|   IBIS file stm32l471_476_ufbga144.ibs
[IBIS ver]   4.2
[File name]   stm32l471_476_ufbga144.ibs
[File Rev]   1.0
[Date]   08-10-2018
[Source]   Data Created at STMicroelectronics
[Notes]   File originated from ELDO simulations.
[Disclaimer]  This information is for modeling purpose only and is
   not guaranteed.
   The information is subject to change without notice.
[Copyright]   Copyright 2018 STMicroelectronics Inc.
|   Component stm32l471_476_ufbga144
[Component] stm32l471_476_ufbga144
[Manufacturer] STMicroelectronics
[Package]
| variable   typ   min   max
R_pkg   0.0   0.0   0.0
L_pkg   0.0H   0.0H   0.0H
C_pkg   0.0F   0.0F   0.0F
[Pin]  signal_name   model_name   R_pin   L_pin   C_pin
A1 VSS GND
A10 PD1 io8prog2m25m50m120m_sudq_ft
A11 PD0 io8prog2m25m50m120m_sudq_ft
A12 VSS GND
A2 PE0 io8prog2m25m50m120m_sudq_ft
A3 PB8 io8prog2m25m50m120m_sudq_i2c_ft
A4 BOOT0 vpp_test_hv
A5 PB7 io8prog2m25m50m120m_sudq_i2c_ft
A6 PG14 io8prog2m25m50m120m_sudq_i2c_ft
A7 PG12 io8prog2m25m50m120m_sudq_ft
A8 PD7 io8prog2m25m50m120m_sudq_ft
A9 PD6 io8prog2m25m50m120m_sudq_ft
B1 VBAT POWER
B10 PC10 io8prog2m25m50m120m_sudq_ft
B11 PA12 io8usblsfs_otg2
B12 PA11 io8usblsfs_otg2
B2 PE4 io8prog2m25m50m120m_sudq_ft
B3 PE3 io8prog2m25m50m120m_sudq_ft
B4 PE1 io8prog2m25m50m120m_sudq_ft
B5 PB6 io8prog2m25m50m120m_sudq_i2c_ft
B6 PG15 io8prog2m25m50m120m_sudq_ft
B7 PG11 io8prog2m25m50m120m_sudq_ft
B8 PD5 io8prog2m25m50m120m_sudq_ft
B9 PC12 io8prog2m25m50m120m_sudq_ft
C1 PC15-OSC32_OUT io8prog2m25m50m120m_sudq_ft
C10 PA14 io8prog2m25m50m120m_sudq_ft
C11 PA13 io8prog2m25m50m120m_sudq_ft
C12 PA10 io8usb_id_otg20_lcd4_ft_ms
C2 PE5 io8prog2m25m50m120m_sudq_ft
C3 PE2 io8prog2m25m50m120m_sudq_ft
C4 PB9 io8prog2m25m50m120m_sudq_i2c_ft
C5 PB5 io8prog2m25m50m120m_sudq_ft
C6 PB3 io8prog2m25m50m120m_sudq_ft
C7 PG9 io8prog2m25m50m120m_sudq_ft
C8 PD4 io8prog2m25m50m120m_sudq_ft
C9 PC11 io8prog2m25m50m120m_sudq_ft
D1 PF4 io8prog2m25m50m120m_sudq_ft
D10 PA15 io8prog2m25m50m120m_sudq_ft
D11 PA9 POWER
D12 PA8 io8prog2m25m50m120m_sudq_ft
D2 PC14-OSC32_IN io8prog2m25m50m120m_sudq_ft
D3 PE6 io8prog2m25m50m120m_sudq_ft
D4 PC13 io8prog2m25m50m120m_sudq_ft
D5 PB4 io8prog2m25m50m120m_sudq_ft
D6 PG13 io8prog2m25m50m120m_sudq_i2c_ft
D7 PG10 io8prog2m25m50m120m_sudq_ft
D8 PD3 io8prog2m25m50m120m_sudq_ft
D9 PD2 io8prog2m25m50m120m_sudq_ft
E1 PF6 io8prog2m25m50m120m_sudq_ft
E10 PC6 io8prog2m25m50m120m_sudq_ft
E11 PC9 io8prog2m25m50m120m_sudq_ft
E12 PC8 io8prog2m25m50m120m_sudq_ft
E2 PF1 io8prog2m25m50m120m_sudq_i2c_ft
E3 PF0 io8prog2m25m50m120m_sudq_i2c_ft
E4 PF2 io8prog2m25m50m120m_sudq_ft
E5 VSS GND
E6 VDDIO2 POWER
E7 VDD POWER
E8 VSS GND
E9 VDD/VDDUSB POWER
F1 PF8 io8prog2m25m50m120m_sudq_ft
F10 PG6 io8prog2m25m50m120m_sudq_ft
F11 PG8 io8prog2m25m50m120m_sudq_i2c_ft
F12 PC7 io8prog2m25m50m120m_sudq_ft
F2 PF7 io8prog2m25m50m120m_sudq_ft
F3 PF5 io8prog2m25m50m120m_sudq_ft
F4 PF3 io8prog2m25m50m120m_sudq_ft
F5 VDD POWER
F6 VSS GND
F7 VSS GND
F8 VDDIO2 POWER
F9 PG7 io8prog2m25m50m120m_sudq_i2c_ft
G1 PH1-OSC_OUT io8prog2m25m50m120m_sudq_ft
G10 PD13 io8prog2m25m50m120m_sudq_ft
G11 PG3 io8prog2m25m50m120m_sudq_ft
G12 PG5 io8prog2m25m50m120m_sudq_ft
G2 PH0-OSC_IN io8prog2m25m50m120m_sudq_ft
G3 PF10 io8prog2m25m50m120m_sudq_ft
G4 PF9 io8prog2m25m50m120m_sudq_ft
G5 VDD POWER
G6 VSS GND
G7 VSS GND
G8 VDD POWER
G9 PG4 io8prog2m25m50m120m_sudq_ft
H1 PC2 io8prog2m25m50m120m_sudq_ft
H10 PD11 io8prog2m25m50m120m_sudq_ft
H11 PD14 io8prog2m25m50m120m_sudq_ft
H12 PG2 io8prog2m25m50m120m_sudq_ft
H2 PC0 io8prog2m25m50m120m_sudq_i2c_ft
H3 PC1 io8prog2m25m50m120m_sudq_i2c_ft
H4 NRST ioreset_ft_v33
H5 VSS GND
H6 VDD POWER
H7 VDD POWER
H8 VSS GND
H9 PD12 io8prog2m25m50m120m_sudq_ft
J1 VSSA GND
J10 PB14 io8prog2m25m50m120m_sudq_i2c_ft
J11 PD10 io8prog2m25m50m120m_sudq_ft
J12 PD15 io8prog2m25m50m120m_sudq_ft
J2 VREF- POWER
J3 PA0 io8prog2m25m50m120m_sudq_ft
J4 PC3 io8prog2m25m50m120m_sudq_ft
J5 PC4 io8prog2m25m50m120m_sudq_ft
J6 PF11 io8prog2m25m50m120m_sudq_ft
J7 PG1 io8prog2m25m50m120m_sudq_ft
J8 PE9 io8prog2m25m50m120m_sudq_ft
J9 PB13 io8prog2m25m50m120m_sudq_i2c_ft
K1 VREF+ POWER
K10 PB12 io8w_swp_lcd4_ft
K11 PD8 io8prog2m25m50m120m_sudq_ft
K12 PD9 io8prog2m25m50m120m_sudq_ft
K2 VDDA POWER
K3 PA1 io8prog2m25m50m120m_sudq_ft
K4 PA6 io8prog2m25m50m120m_sudq_ft
K5 PB2 io8prog2m25m50m120m_sudq_ft
K6 PF12 io8prog2m25m50m120m_sudq_ft
K7 PG0 io8prog2m25m50m120m_sudq_ft
K8 PE11 io8prog2m25m50m120m_sudq_ft
K9 PB11 io8prog2m25m50m120m_sudq_i2c_ft
L1 OPAMP1_VINM NC
L10 PE14 io8prog2m25m50m120m_sudq_ft
L11 PB10 io8prog2m25m50m120m_sudq_i2c_ft
L12 PB15 io8prog2m25m50m120m_sudq_ft
L2 PA2 io8prog2m25m50m120m_sudq_ft
L3 PA4 io8prog2m25m50m120m_sudq_ft
L4 OPAMP2_VINM NC
L5 PB0 io8prog2m25m50m120m_sudq_ft
L6 PF13 io8prog2m25m50m120m_sudq_ft
L7 PE8 io8prog2m25m50m120m_sudq_ft
L8 PE12 io8prog2m25m50m120m_sudq_ft
L9 PE13 io8prog2m25m50m120m_sudq_ft
M1 VSS GND
M10 PE10 io8prog2m25m50m120m_sudq_ft
M11 PE15 io8prog2m25m50m120m_sudq_ft
M12 VSS GND
M2 PA3 io8prog2m25m50m120m_sudq_ft
M3 PA5 io8prog2m25m50m120m_sudq_ft
M4 PA7 io8prog2m25m50m120m_sudq_ft
M5 PC5 io8prog2m25m50m120m_sudq_ft
M6 PB1 io8prog2m25m50m120m_sudq_ft
M7 PF14 io8prog2m25m50m120m_sudq_ft
M8 PE7 io8prog2m25m50m120m_sudq_ft
M9 PF15 io8prog2m25m50m120m_sudq_ft
[Model Selector] io8prog2m25m50m120m_sudq_ft
iols8p_sudq_ft_pd_lv  "IO low speed, PD=40kOhm - 1P8V"
iols8p_sudq_ft_pu_lv  "IO low speed, PU=40kOhm - 1P8V"
iols8p_sudq_ft_lv  "IO low speed - 1P8V"
iols8p_sudq_ft_pd  "IO low speed, PD=40kOhm - 3P3V"
iols8p_sudq_ft_pu  "IO low speed, PU=40kOhm - 3P3V"
iols8p_sudq_ft  "IO low speed - 3P3V"
iofs8p_sudq_ft_pd_lv  "IO full speed, PD=40kOhm - 1P8V"
iofs8p_sudq_ft_pu_lv  "IO full speed, PU=40kOhm - 1P8V"
iofs8p_sudq_ft_lv  "IO full speed - 1P8V"
iofs8p_sudq_ft_pd  "IO full speed, PD=40kOhm - 3P3V"
iofs8p_sudq_ft_pu  "IO full speed, PU=40kOhm - 3P3V"
iofs8p_sudq_ft  "IO full speed - 3P3V"
ioms8p_sudq_ft_pd_lv  "IO medium speed, PD=40kOhm - 1P8V"
ioms8p_sudq_ft_pu_lv  "IO medium speed, PU=40kOhm - 1P8V"
ioms8p_sudq_ft_lv  "IO medium speed - 1P8V"
ioms8p_sudq_ft_pd  "IO medium speed, PD=40kOhm - 3P3V"
ioms8p_sudq_ft_pu  "IO medium speed, PU=40kOhm - 3P3V"
ioms8p_sudq_ft  "IO medium speed - 3P3V"
iohs8p_sudq_ft_pd_lv  "IO high speed, PD=40kOhm - 1P8V"
iohs8p_sudq_ft_pu_lv  "IO high speed, PU=40kOhm - 1P8V"
iohs8p_sudq_ft_lv  "IO high speed - 1P8V"
iohs8p_sudq_ft_pd  "IO high speed, PD=40kOhm - 3P3V"
iohs8p_sudq_ft_pu  "IO high speed, PU=40kOhm - 3P3V"
iohs8p_sudq_ft  "IO high speed - 3P3V"
[Model Selector] io8prog2m25m50m120m_sudq_i2c_ft
io8prog_1v8_i2c_pd  "5V Tol GPIO 1.8V range i2c functionality with pull down"
io8prog_1v8_i2c_pu  "5V Tol GPIO 1.8V range i2c functionality with pull up"
io8prog_1v8_i2c  "5V Tol GPIO 1.8V range i2c functionality"
io8prog_3v3_i2c_pd  "5V Tol GPIO 3.3V range i2c functionality with pull down"
io8prog_3v3_i2c_pu  "5V Tol GPIO 3.3V range i2c functionality with pull up"
io8prog_3v3_i2c  "5V Tol GPIO 3.3V range i2c functionality"
io8ls_1v8_pd  "5V Tol GPIO 1.8V range with pd io low speed"
io8ls_1v8_pu  "5V Tol GPIO 1.8V range with pu io low speed"
io8ls_1v8  "5V Tol GPIO 1.8V range io low speed"
io8ls_3v3_pd  "5V Tol GPIO 3.3V range with pd io low speed"
io8ls_3v3_pu  "5V Tol GPIO 3.3V range with pu io low speed"
io8ls_3v3  "5V Tol GPIO 3.3V range io low speed"
io8fs_1v8_pd  "5V Tol GPIO 1.8V range with pd io full speed"
io8fs_1v8_pu  "5V Tol GPIO 1.8V range with pu io full speed"
io8fs_1v8  "5V Tol GPIO 1.8V range io full speed"
io8fs_3v3_pd  "5V Tol GPIO 3.3V range with pd io full speed"
io8fs_3v3_pu  "5V Tol GPIO 3.3V range with pu io full speed"
io8fs_3v3  "5V Tol GPIO 3.3V range io full speed"
io8ms_1v8_pd  "5V Tol GPIO 1.8V range with pd io medium speed"
io8ms_1v8_pu  "5V Tol GPIO 1.8V range with pu io medium speed"
io8ms_1v8  "5V Tol GPIO 1.8V range io medium speed"
io8ms_3v3_pd  "5V Tol GPIO 3.3V range with pd io medium speed"
io8ms_3v3_pu  "5V Tol GPIO 3.3V range with pu io medium speed"
io8ms_3v3  "5V Tol GPIO 3.3V range io medium speed"
io8hs_1v8_pd  "5V Tol GPIO 1.8V range with pd io high speed"
io8hs_1v8_pu  "5V Tol GPIO 1.8V range with pu io high speed"
io8hs_1v8  "5V Tol GPIO 1.8V range io high speed"
io8hs_3v3_pd  "5V Tol GPIO 3.3V range with pd io high speed"
io8hs_3v3_pu  "5V Tol GPIO 3.3V range with pu io high speed"
io8hs_3v3  "5V Tol GPIO 3.3V range io high speed"
[Model Selector] io8usb_id_otg20_lcd4_ft_ms
io8usbid_1v8_id_pu  "ID 1V8 range with pull up"
io8usbid_3v3_id_pu  "ID 3V3 range with pull up"
io8usbid_1v8_id  "ID 1V8 range"
io8usbid_3v3_id  "ID 3V3 range"
io8lsusbid_1v8_pd  "GPIO 1.8V range with pd io low speed"
io8lsusbid_1v8_pu  "GPIO 1.8V range with pu io low speed"
io8lsusbid_1v8  "GPIO 1.8V range io low speed"
io8lsusbid_3v3_pd  "GPIO 3.3V range with pd io low speed"
io8lsusbid_3v3_pu  "GPIO 3.3V range with pu io low speed"
io8lsusbid_3v3  "GPIO 3.3V range io low speed"
io8fsusbid_1v8_pd  "GPIO 1.8V range with pd io full speed"
io8fsusbid_1v8_pu  "GPIO 1.8V range with pu io full speed"
io8fsusbid_1v8  "GPIO 1.8V range io full speed"
io8fsusbid_3v3_pd  "GPIO 3.3V range with pd io full speed"
io8fsusbid_3v3_pu  "GPIO 3.3V range with pu io full speed"
io8fsusbid_3v3  "GPIO 3.3V range io full speed"
io8msusbid_1v8_pd  "GPIO 1.8V range with pd io medium speed"
io8msusbid_1v8_pu  "GPIO 1.8V range with pu io medium speed"
io8msusbid_1v8  "GPIO 1.8V range io medium speed"
io8msusbid_3v3_pd  "GPIO 3.3V range with pd io medium speed"
io8msusbid_3v3_pu  "GPIO 3.3V range with pu io medium speed"
io8msusbid_3v3  "GPIO 3.3V range io medium speed"
io8hsusbid_1v8_pd  "GPIO 1.8V range with pd io high speed"
io8hsusbid_1v8_pu  "GPIO 1.8V range with pu io high speed"
io8hsusbid_1v8  "GPIO 1.8V range io high speed"
io8hsusbid_3v3_pd  "GPIO 3.3V range with pd io high speed"
io8hsusbid_3v3_pu  "GPIO 3.3V range with pu io high speed"
io8hsusbid_3v3  "GPIO 3.3V range io high speed"
[Model Selector] io8usblsfs_otg2
usb_ls_pd  "USB Low Speed mode - Pull Down"
usb_ls_pu2  "USB Low Speed mode - Pull up 2"
usb_ls_pu  "USB Low Speed mode - Pull up"
usb_fs  "USB Low Speed mode"
usb_fs_pd  "USB Full Speed mode - Pull Down"
usb_fs_pu2  "USB Full Speed mode - Pull up 2"
usb_fs_pu  "USB Full Speed mode - Pull up"
[Model Selector] ioreset_ft_v33
ioreset_1v2_pu  "RESET 1.2V range with PU"
ioreset_1v2  "RESET 1.2V range"
ioreset_1v8_pu  "RESET 1.8V range with PU"
ioreset_1v8  "RESET 1.8V range"
ioreset_3v3_pu  "RESET 3.3V range with PU"
ioreset_3v3  "RESET 3.3V range"
[Model Selector] io8w_swp_lcd4_ft
io8w_swp_classc  "Class C swp functionality"
io8w_swp_classb  "Class B swp functionality"
io8lsw_1v8_pd  "GPIO 1.8V range with pd io low speed"
io8lsw_1v8_pu  "GPIO 1.8V range with pu io low speed"
io8lsw_1v8  "GPIO 1.8V range io low speed"
io8lsw_3v3_pd  "GPIO 3.3V range with pd io low speed"
io8lsw_3v3_pu  "GPIO 3.3V range with pu io low speed"
io8lsw_3v3  "GPIO 3.3V range io low speed"
io8fsw_1v8_pd  "GPIO 1.8V range with pd io full speed"
io8fsw_1v8_pu  "GPIO 1.8V range with pu io full speed"
io8fsw_1v8  "GPIO 1.8V range io full speed"
io8fsw_3v3_pd  "GPIO 3.3V range with pd io full speed"
io8fsw_3v3_pu  "GPIO 3.3V range with pu io full speed"
io8fsw_3v3  "GPIO 3.3V range io full speed"
io8msw_1v8_pd  "GPIO 1.8V range with pd io medium speed"
io8msw_1v8_pu  "GPIO 1.8V range with pu io medium speed"
io8msw_1v8  "GPIO 1.8V range io medium speed"
io8msw_3v3_pd  "GPIO 3.3V range with pd io medium speed"
io8msw_3v3_pu  "GPIO 3.3V range with pu io medium speed"
io8msw_3v3  "GPIO 3.3V range io medium speed"
io8hsw_1v8_pd  "GPIO 1.8V range with pd io high speed"
io8hsw_1v8_pu  "GPIO 1.8V range with pu io high speed"
io8hsw_1v8  "GPIO 1.8V range io high speed"
io8hsw_3v3_pd  "GPIO 3.3V range with pd io high speed"
io8hsw_3v3_pu  "GPIO 3.3V range with pu io high speed"
io8hsw_3v3  "GPIO 3.3V range io high speed"
[Model Selector] vpp_test_hv
vpp_1v8  "VPP with test functionality 1.8V range"
vpp_3v3  "VPP with test functionality 3.3V range"
| Models and submodels in the file (123): iols8p_sudq_ft_pd_lv (I/O), iols8p_sudq_ft_pu_lv (I/O), iols8p_sudq_ft_lv (I/O), iols8p_sudq_ft_pd (I/O), iols8p_sudq_ft_pu (I/O), iols8p_sudq_ft (I/O), iofs8p_sudq_ft_pd_lv (I/O), iofs8p_sudq_ft_pu_lv (I/O), iofs8p_sudq_ft_lv (I/O), iofs8p_sudq_ft_pd (I/O), iofs8p_sudq_ft_pu (I/O), iofs8p_sudq_ft (I/O), ioms8p_sudq_ft_pd_lv (I/O), ioms8p_sudq_ft_pu_lv (I/O), ioms8p_sudq_ft_lv (I/O), ioms8p_sudq_ft_pd (I/O), ioms8p_sudq_ft_pu (I/O), ioms8p_sudq_ft (I/O), iohs8p_sudq_ft_pd_lv (I/O), iohs8p_sudq_ft_pu_lv (I/O), iohs8p_sudq_ft_lv (I/O), iohs8p_sudq_ft_pd (I/O), iohs8p_sudq_ft_pu (I/O), iohs8p_sudq_ft (I/O), io8prog_1v8_i2c_pd (I/O), io8prog_1v8_i2c_pu (I/O), io8prog_1v8_i2c (I/O), io8prog_3v3_i2c_pd (I/O), io8prog_3v3_i2c_pu (I/O), io8prog_3v3_i2c (I/O), io8ls_1v8_pd (I/O), io8ls_1v8_pu (I/O), io8ls_1v8 (I/O), io8ls_3v3_pd (I/O), io8ls_3v3_pu (I/O), io8ls_3v3 (I/O), io8fs_1v8_pd (I/O), io8fs_1v8_pu (I/O), io8fs_1v8 (I/O), io8fs_3v3_pd (I/O), io8fs_3v3_pu (I/O), io8fs_3v3 (I/O), io8ms_1v8_pd (I/O), io8ms_1v8_pu (I/O), io8ms_1v8 (I/O), io8ms_3v3_pd (I/O), io8ms_3v3_pu (I/O), io8ms_3v3 (I/O), io8hs_1v8_pd (I/O), io8hs_1v8_pu (I/O), io8hs_1v8 (I/O), io8hs_3v3_pd (I/O), io8hs_3v3_pu (I/O), io8hs_3v3 (I/O), io8usbid_1v8_id_pu (Input), io8usbid_3v3_id_pu (Input), io8usbid_1v8_id (Input), io8usbid_3v3_id (Input), io8lsusbid_1v8_pd (I/O), io8lsusbid_1v8_pu (I/O), io8lsusbid_1v8 (I/O), io8lsusbid_3v3_pd (I/O), io8lsusbid_3v3_pu (I/O), io8lsusbid_3v3 (I/O), io8fsusbid_1v8_pd (I/O), io8fsusbid_1v8_pu (I/O), io8fsusbid_1v8 (I/O), io8fsusbid_3v3_pd (I/O), io8fsusbid_3v3_pu (I/O), io8fsusbid_3v3 (I/O), io8msusbid_1v8_pd (I/O), io8msusbid_1v8_pu (I/O), io8msusbid_1v8 (I/O), io8msusbid_3v3_pd (I/O), io8msusbid_3v3_pu (I/O), io8msusbid_3v3 (I/O), io8hsusbid_1v8_pd (I/O), io8hsusbid_1v8_pu (I/O), io8hsusbid_1v8 (I/O), io8hsusbid_3v3_pd (I/O)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
